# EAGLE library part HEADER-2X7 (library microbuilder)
PIN HEADER
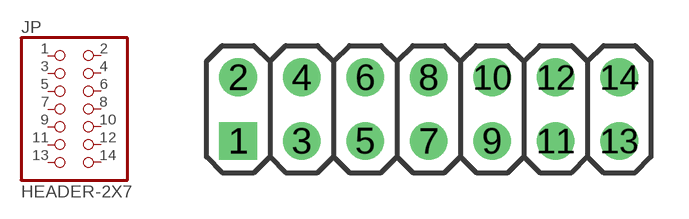
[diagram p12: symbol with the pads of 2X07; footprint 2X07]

Designator prefix JP

## HEADER-2X7  [2X07]
1  1  pas
2  2  pas
3  3  pas
4  4  pas
5  5  pas
6  6  pas
7  7  pas
8  8  pas
9  9  pas
10  10  pas
11  11  pas
12  12  pas
13  13  pas
14  14  pas

## Footprint 2X07 (pad centres in mm)
PIN HEADER
drill 1 square: 1 -7.62,-1.27
drill 1: 2 -7.62,1.27; 3 -5.08,-1.27; 4 -5.08,1.27; 5 -2.54,-1.27; 6 -2.54,1.27; 7 0,-1.27; 8 0,1.27; 9 2.54,-1.27; 10 2.54,1.27; 11 5.08,-1.27; 12 5.08,1.27; 13 7.62,-1.27; 14 7.62,1.27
